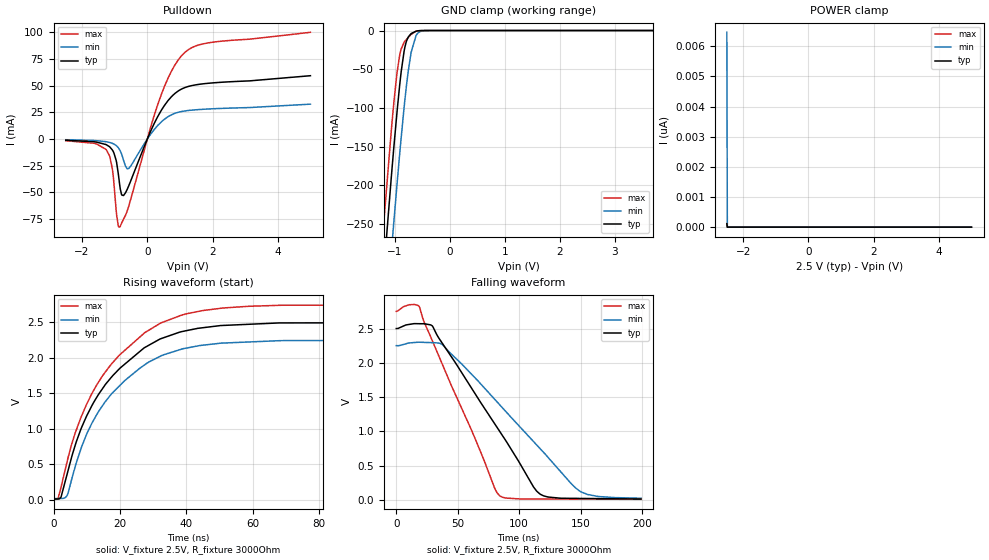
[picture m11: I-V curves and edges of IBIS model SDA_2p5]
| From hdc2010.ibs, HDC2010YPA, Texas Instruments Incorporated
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[Model]   SDA_2p5
Model_type   I/O_open_drain
Polarity   Non-Inverting
Enable   Active-Low
Vinl = 0.75
Vinh = 1.75
Vmeas = 1.25
Vref = 2.5
Cref = 15pF
Rref = 3000
|   typ   min   max
|   (nom PVT)   (slow PVT)   (fast PVT)
C_comp   1.615p   1.567p   1.665p
|C_comp (ON state)   1.615p   1.567p   1.665p
|C_comp (OFF state)   1.835p   1.693p   1.938p
[Model spec]
|subparameter
Vinl   0.75   0.675   0.825
Vinh   1.75   1.575   1.925
[Voltage Range]   2.5   2.25   2.75
[Temperature Range]   27   125   -40
[Pullup Reference]   2.5   2.25   2.75
[Pulldown Reference]   0   -0   -0
[Power Clamp Reference]   2.5   2.25   2.75
[GND Clamp Reference]   0   0   0
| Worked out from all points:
|   slope of the pulldown table from 0 to 0.375 V, typ, clamps not added: 15.6 ohm
|   GND clamp passes 1 mA (typ) near -0.62 V on its own axis
|   falling waveform, V_fixture 2.5V, R_fixture 3000Ohm: 20-80 % time 53.2ns typ, 68.1ns min, 39.7ns max; typ from 2.5 V to 0.012 V
|   rising waveform, V_fixture 2.5V, R_fixture 3000Ohm: 20-80 % time 18.9ns typ, 18.2ns min, 19.6ns max; typ from 0.01 V to 2.5 V
[Pulldown]
|   Voltage   I(typ)   I(min)   I(max)
-2.5V     -1.129mA   -659.3uA   -1.599mA
-1.255V   -5.381mA   -2.568mA   -10.19mA
-1.075V   -10.13mA   -4.02mA    -27.43mA
-940mV    -22.32mA   -6.491mA   -71.62mA
-850mV    -42.22mA   -9.97mA    -82.69mA
-730mV    -53.02mA   -19.78mA   -75.23mA
-572.5mV  -44.13mA   -27.65mA   -63.26mA
327.5mV   21.51mA    12.98mA    33.05mA
732.5mV   39.45mA    22.62mA    63.21mA
1.093V    47.51mA    26.05mA    79.52mA
1.798V    52.08mA    28.05mA    89.82mA
5V        59.4mA     32.71mA    100.1mA
[GND Clamp]
|   Voltage   I(typ)   I(min)   I(max)
-2.5V     -1.554A    -1.646A    -1.496A
-1.225V   -328.2mA   -426.9mA   -265mA
-1.067V   -188.7mA   -286.1mA   -128.4mA
-1.045V   -169.7mA   -266.6mA   -110.6mA
-1.03V    -157.2mA   -253.7mA   -99.09mA
-962.5mV  -103.8mA   -197mA     -53.75mA
-917.5mV  -71.65mA   -160.7mA   -32.59mA
-835mV    -26.6mA    -99.2mA    -15.26mA
-707.5mV  -3.922mA   -28.18mA   -5.038mA
-617.5mV  -838uA     -6.457mA   -914.2uA
-392.5mV  -2.28uA    -54.26uA   -330nA
5V        0A         0A         0A
[POWER Clamp]
|   Voltage   I(typ)   I(min)   I(max)
-2.5V     120pA      6.462nA    105.4pA
-2.485V   0A         0A         0A
-2.478V   0A         0A         0A
5V        0A         0A         0A
[Ramp]
R_load = 3000
|   typ   min   max
dV/dt_r   1.49383/1.87712e-08   1.34076/1.81775e-08   1.64687/1.95203e-08
dV/dt_f   1.49298/5.32389e-08   1.33578/6.81388e-08   1.64541/3.96479e-08
[Falling Waveform]
V_fixture = 2.5V
V_fixture_min = 2.25V
V_fixture_max = 2.75V
R_fixture = 3000Ohm
C_fixture = 0F
|   Time   V(typ)   V(min)   V(max)
0s        2.5V       2.25V      2.75V
10.2ns    2.559V     2.289V     2.846V
18.62ns   2.571V     2.301V     2.822V
29.26ns   2.539V     2.294V     2.324V
37.29ns   2.288V     2.268V     1.984V
84.01ns   1.001V     1.389V     60.55mV
111.7ns   186.7mV    849.8mV    12.65mV
119.8ns   58.26mV    692.5mV    12.16mV
150.5ns   20.33mV    114.4mV    10.33mV
199ns     11.69mV    23.69mV    7.442mV
[Rising Waveform]
V_fixture = 2.5V
V_fixture_min = 2.25V
V_fixture_max = 2.75V
R_fixture = 3000Ohm
C_fixture = 0F
|   Time   V(typ)   V(min)   V(max)
0s        10.28mV    15.33mV    5.219mV
1.425ns   10.41mV    16.67mV    28.97mV
2.217ns   32.9mV     17.42mV    168.3mV
4.121ns   365.2mV    61.87mV    541.6mV
8.399ns   1.013V     738.3mV    1.175V
14.77ns   1.567V     1.326V     1.747V
25.96ns   2.088V     1.852V     2.291V
38.53ns   2.367V     2.121V     2.6V
68.58ns   2.49V      2.241V     2.739V
199ns     2.5V       2.25V      2.75V
